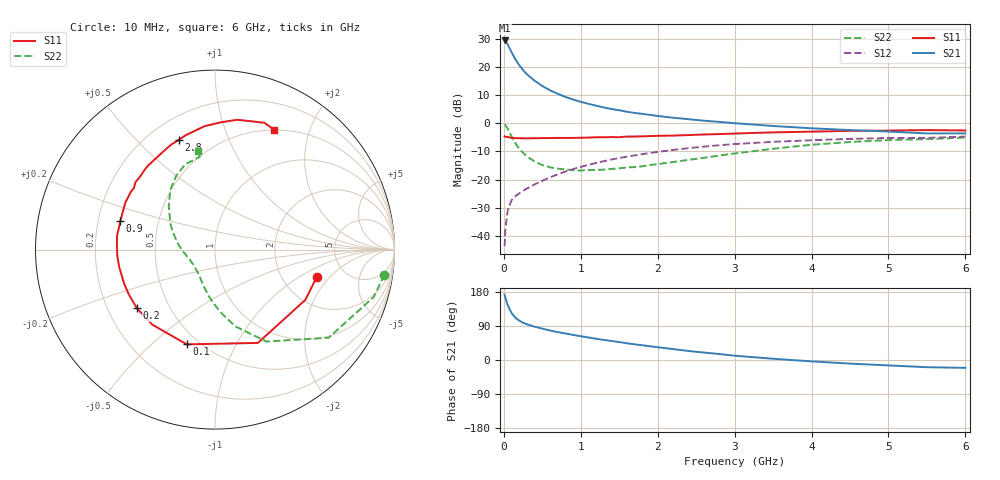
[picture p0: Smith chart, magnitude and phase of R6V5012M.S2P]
! SIEMENS Small Signal Semiconductors
! BFR193
! Si NPN RF Bipolar Junction Transistor in SOT23
! VCE = 0.5 V  IC = 12 mA
! Common Emitter S-Parameters:  May  1996
# GHz  S  MA  R  50
!  f  S11  S21  S12  S22
! GHz  MAG  ANG  MAG  ANG  MAG  ANG  MAG  ANG
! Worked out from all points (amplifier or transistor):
!   36 points, 10 MHz to 6 GHz, reference 50 ohm
!   highest |S21| = 29.4 dB at 10 MHz (marker M1)
!   |S21| within 3 dB of that: start of sweep to 79.13 MHz
!   unconditionally stable (mu >= 1): 590.3 MHz to 2.539 GHz
!   at 250 MHz: K = 0.72, MSG = 21.4 dB, |S12| = -24.0 dB
!   at 1.4 GHz: K = 1.06, MAG = 7.5 dB, |S12| = -12.9 dB
!   at 6 GHz: K = 1.00, MSG = 0.6 dB, |S12| = -4.7 dB
!   S11 on the Smith chart (normalised r, x): 10 MHz: 3.13, -1.44; 100 MHz: 0.43, -0.65; 200 MHz: 0.32, -0.30; 900 MHz: 0.30, +0.13; 2.8 GHz: 0.32, +0.67; 6 GHz: 0.50, +1.49
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0.01  0.5879 -14.9  29.5 172.3  0.0066 82.5  0.9538 -8.4
0.02  0.576 -29.1  28.92 164.4  0.0133 78.4  0.9231 -16.6
0.05  0.5722 -65.3  25.11 145.0  0.0283 64.1  0.8012 -37.8
0.1  0.551 -106.6  18.3 124.0  0.043 52.9  0.5868 -60.8
0.15  0.5447 -129.9  13.66 111.5  0.0508 50.1  0.4417 -75.3
0.2  0.5442 -143.1  10.77 104.0  0.0572 49.8  0.3557 -84.3
0.25  0.5413 -152.9  8.783 98.3  0.0634 50.8  0.2978 -91.9
0.3  0.5406 -159.8  7.421 94.2  0.0696 52.6  0.2579 -98.2
0.4  0.5428 -170.0  5.689 88.0  0.0823 55.2  0.21 -108.1
0.5  0.5455 -176.6  4.586 82.8  0.0955 57.0  0.1815 -116.1
0.6  0.5472 177.1  3.857 77.9  0.1099 58.3  0.1659 -123.3
0.7  0.551 172.0  3.343 73.6  0.1243 58.8  0.1568 -129.9
0.9  0.5505 163.4  2.64 66.3  0.154 58.5  0.1467 -140.9
1.1  0.5575 155.9  2.213 59.4  0.1831 57.3  0.1477 -149.0
1.3  0.5647 149.1  1.909 53.0  0.2128 55.4  0.1505 -157.7
1.6  0.5809 139.7  1.602 44.2  0.2559 51.9  0.1646 -168.8
2.2  0.6051 123.3  1.254 28.8  0.3373 43.3  0.2053 172.2
2.8  0.6433 108.4  1.059 15.8  0.4074 33.9  0.2679 154.2
3.5  0.6903 94.8  0.895 3.3  0.4687 22.6  0.3534 136.8
4.5  0.7337 80.3  0.758 -9.5  0.5288 8.6  0.4657 117.5
5.5  0.7583 68.7  0.661 -19.0  0.5508 -4.5  0.5237 99.3
6  0.7451 63.8  0.662 -20.7  0.5816 -8.4  0.5586 100.0
